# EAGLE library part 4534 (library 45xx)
BCD COUNTER
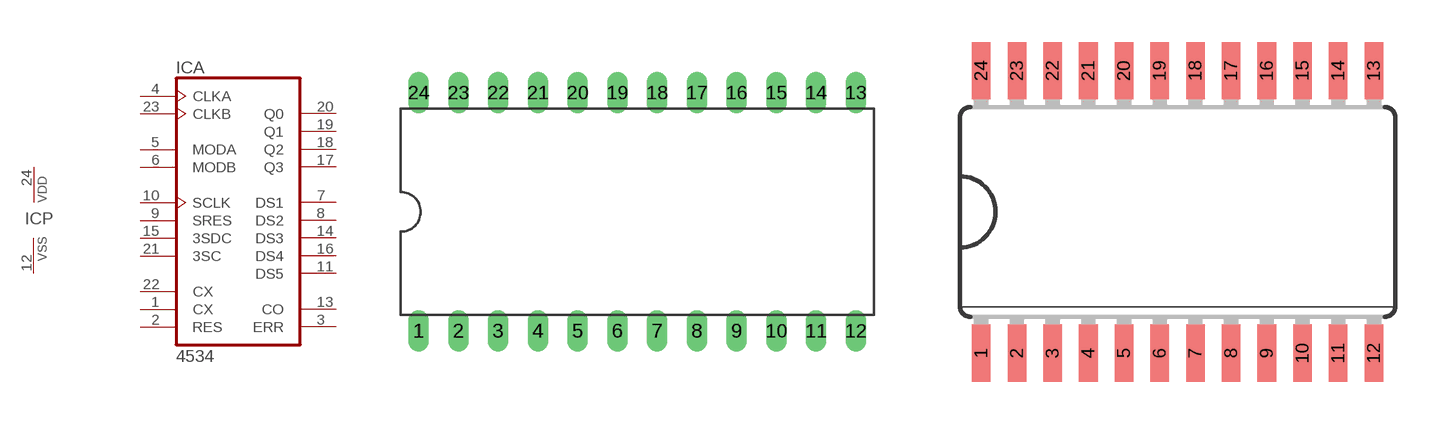
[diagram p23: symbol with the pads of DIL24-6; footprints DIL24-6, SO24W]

Designator prefix IC; gates A=4534 P=PWRN

## 4534N  [DIL24-6]
1  A:CX  in
2  A:RES  in
3  A:ERR  out
4  A:CLKA  in
5  A:MODA  in
6  A:MODB  in
7  A:DS1  hiz
8  A:DS2  hiz
9  A:SRES  in
10  A:SCLK  in
11  A:DS5  hiz
12  P:VSS  pwr
13  A:CO  out
14  A:DS3  hiz
15  A:3SDC  in
16  A:DS4  hiz
17  A:Q3  hiz
18  A:Q2  hiz
19  A:Q1  hiz
20  A:Q0  hiz
21  A:3SC  in
22  A:CX  in
23  A:CLKB  in
24  P:VDD  pwr

## 4534D  [SO24W]
Pads as for DIL24-6

## Footprint DIL24-6 (pad centres in mm)
Dual In Line Package 0.6 inch
drill 0.813 long: 1 -13.97,-7.62; 2 -11.43,-7.62; 3 -8.89,-7.62; 4 -6.35,-7.62; 5 -3.81,-7.62; 6 -1.27,-7.62; 7 1.27,-7.62; 8 3.81,-7.62; 9 6.35,-7.62; 10 8.89,-7.62; 11 11.43,-7.62; 12 13.97,-7.62; 13 13.97,7.62; 14 11.43,7.62; 15 8.89,7.62; 16 6.35,7.62; 17 3.81,7.62; 18 1.27,7.62; 19 -1.27,7.62; 20 -3.81,7.62; 21 -6.35,7.62; 22 -8.89,7.62; 23 -11.43,7.62; 24 -13.97,7.62

## Footprint SO24W (pad centres in mm)
Wide Small Outline package 300 mil
smd 0.66 x 2.032: 1 -6.985,-5.029; 2 -5.715,-5.029; 3 -4.445,-5.029; 4 -3.175,-5.029; 5 -1.905,-5.029; 6 -0.635,-5.029; 7 0.635,-5.029; 8 1.905,-5.029; 9 3.175,-5.029; 10 4.445,-5.029; 11 5.715,-5.029; 12 6.985,-5.029; 13 6.985,5.029; 14 5.715,5.029; 15 4.445,5.029; 16 3.175,5.029; 17 1.905,5.029; 18 0.635,5.029; 19 -0.635,5.029; 20 -1.905,5.029; 21 -3.175,5.029; 22 -4.445,5.029; 23 -5.715,5.029; 24 -6.985,5.029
